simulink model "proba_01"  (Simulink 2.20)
settings: Solver=ode45  StartTime=0.0  StopTime=39.9  RelTol=1e-3  AbsTol=1e-6
libraries: simulink x1

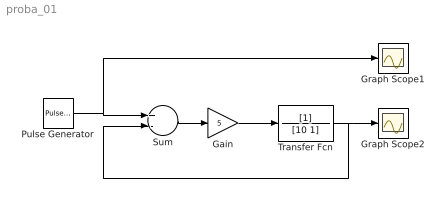
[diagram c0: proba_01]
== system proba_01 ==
  Gain : Gain  Gain=5
  Graph Scope1 : Scope
  Graph Scope2 : Scope
  Pulse Generator : simulink/Sources/Pulse Generator  period=40  duty=50  amplitude=1  start=0
  Sum : Sum  Inputs=+-
  Transfer Fcn : TransferFcn  Numerator=[1]  Denominator=[10 1]
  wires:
  Sum/1 -> Gain/1
  Gain/1 -> Transfer Fcn/1
  Pulse Generator/1 -> Sum/1, Graph Scope1/1
  Transfer Fcn/1 -> Graph Scope2/1, Sum/2
